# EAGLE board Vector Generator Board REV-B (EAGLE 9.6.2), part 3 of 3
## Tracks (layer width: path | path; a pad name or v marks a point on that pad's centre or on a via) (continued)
XBRM5 (continued)
  Top 0.381: 8C/8D.3 188.59,186.69 188.59,173.74 182.5,167.64 7D.12
XBRM6  (via drill 0.35)
  Top 0.381: v192.79,164.97 182.5,164.97 7D.11
  Bottom 0.381: v192.79,164.97 192.79,150.5 194.69,148.59 8D/8E.4
XBRM7  (via drill 0.35)
  Top 0.381: v174.88,155.83 175.26,156.21 184.4,156.21 | 8D/8E.1 184.4,156.21 | 7D.10 184.4,160.4 184.4,156.21
  Bottom 0.381: v174.88,155.83 174.88,137.16 7E.1
XBRM8
  Top 0.381: 7E.13 192.41,144.78 196.22,144.78 196.98,145.54 196.98,150.88 202.31,150.88 8D/8E.14
XBRM9
  Top 0.381: 7E.12 182.5,132.21 187.45,137.16 196.22,137.16 200.41,141.35 200.41,144.78 203.84,144.78 204.6,145.54 204.6,153.54 202.69,153.54 8D/8E.15
XBRM10
  Top 0.381: 7E.11 182.12,129.54 180.21,131.44 180.21,153.54 194.69,153.54 8D/8E.2
XBRM11  (via drill 0.35)
  Top 0.381: v189.74,127.25 182.5,127.25 7E.10 182.12,127.25 176.02,133.35 172.97,133.35 164.59,141.73 129.54,141.73 v128.78,142.49 | v189.74,150.88 194.69,150.88 8D/8E.3 | v40.39,238.51 52.58,238.51 1B.3 | v87.63,147.83 v40.39,147.83 | v87.63,151.26 102.87,151.26 104.39,152.78 107.82,152.78 113.54,158.5 v128.78,158.5
  Bottom 0.381: v189.74,150.88 v189.74,127.25 | v40.39,147.83 v40.39,238.51 | v87.63,151.26 v87.63,147.83 | v128.78,142.49 v128.78,158.5
XBRMRATE  (via drill 0.35)
  Top 0.381: v187.45,280.42 185.17,278.13 176.02,278.13 174.88,276.99 7A.2 | v192.79,187.83 v187.45,187.83
  Bottom 0.381: v187.45,187.83 v187.45,280.42 | v192.79,187.83 192.79,180.97 194.69,179.07 8C/8D.6
XCUR0  (via drill 0.35)
  Top 0.381: v70.87,230.12 67.06,226.31 55.25,226.31 51.05,222.12 46.48,222.12 45.72,221.36 45.72,214.5 66.68,214.5 | 66.68,214.5 75.44,214.5 80.39,209.55 2C.19 | v128.78,182.5 v161.93,182.5 | v128.78,164.21 128.4,164.59 116.21,164.59 104.78,176.02 v67.82,176.02 | v67.82,212.22 67.44,212.22 66.68,212.98 66.68,214.5
  Bottom 0.381: v70.87,230.12 70.87,241.94 72.77,243.84 2B.1 | v161.93,182.5 6C.9 | v128.78,164.21 v128.78,182.5 | v67.82,212.22 v67.82,176.02
XCUR1  (via drill 0.35)
  Top 0.381: 2C.18 74.3,213.36 v67.82,213.36 | 70.87,238.51 72.77,238.51 2B.3 | 70.87,238.51 v67.82,238.51 | v127.64,181.36 v163.83,181.36 | v116.21,208.41 v127.64,208.41 | v115.06,216.03 114.68,215.65 96.01,215.65 95.63,216.03 92.58,216.03 87.25,221.36 v87.25,221.74 | v87.25,245.36 72.01,245.36 70.87,244.22 70.87,238.51
  Bottom 0.381: v67.82,238.51 v67.82,213.36 | v163.83,181.36 163.83,195.83 162.69,195.83 161.93,196.6 6C.11 | v127.64,208.41 v127.64,181.36 | v116.21,208.41 116.21,214.5 115.06,215.65 v115.06,216.03 | v87.25,245.36 v87.25,221.74
XCUR2  (via drill 0.35)
  Top 0.381: v78.11,224.03 v75.06,224.03 | v159.26,213.74 139.06,213.74 137.16,215.65 116.59,215.65 v116.21,216.03 | v116.21,221.36 115.82,220.98 105.54,220.98 102.87,223.65 83.06,223.65 v81.92,224.79
  Bottom 0.381: 2B.5 75.06,231.65 v75.06,224.03 | 78.11,221.74 78.11,206.88 80.39,204.6 2C.17 | 78.11,221.74 v78.11,224.03 | v159.26,213.74 159.26,206.12 160.4,204.98 160.4,204.6 161.93,204.6 6C.14 | v116.21,221.36 v116.21,216.03 | v81.92,224.79 80.39,223.27 80.39,222.5 79.63,221.74 78.11,221.74
XCUR3  (via drill 0.35)
  Top 0.381: v75.82,203.07 79.25,203.07 80.39,201.93 2C.16 | v79.25,222.88 v75.82,222.88 | v154.31,217.17 129.92,217.17 128.4,218.69 112.01,218.69 v111.63,218.31 | v112.01,228.6 103.63,228.6 102.11,227.08 84.58,227.08 80.77,230.89 2B.9
  Bottom 0.381: v75.82,222.88 v75.82,203.07 | v79.25,222.88 79.25,227.46 78.49,228.22 78.49,228.98 2B.9 | v154.31,217.17 6C.1 | v111.63,218.31 112.01,218.69 v112.01,228.6
XCUR4  (via drill 0.35)
  Top 0.381: v65.53,198.12 74.3,198.12 75.06,198.88 80.01,198.88 80.39,199.26 2C.15 | v65.53,231.65 65.91,232.03 71.25,232.03 71.63,232.41 76.58,232.41 80.39,236.22 2B.11 | 6D.9 159.26,153.54 v143.64,153.54 | v143.64,167.64 119.63,167.64 v119.25,168.02 | v116.97,171.83 115.06,173.74 110.87,173.74 105.16,179.45 v65.53,179.45
  Bottom 0.381: v65.53,231.65 v65.53,198.12 v65.53,179.45 | v143.64,167.64 v143.64,153.54 | v119.25,168.02 116.97,170.31 v116.97,171.83
XCUR5  (via drill 0.35)
  Top 0.381: v148.97,160.02 155.45,160.02 156.21,160.78 161.54,160.78 161.93,161.16 6D.11 | v148.97,214.88 139.06,214.88 137.54,216.41 129.54,216.41 128.02,217.93 112.78,217.93 112.01,217.17 99.06,217.17 96.01,220.22 v94.87,220.22 | v95.25,232.03 94.87,232.41 v82.68,232.41
  Bottom 0.381: 2B.13 82.68,239.27 v82.68,232.41 79.25,232.41 77.72,230.89 77.72,225.55 76.96,224.79 76.96,200.41 80.39,196.98 2C.14 | v148.97,214.88 v148.97,160.02 | v94.87,220.22 94.87,227.46 95.25,227.84 v95.25,232.03
XCUR6  (via drill 0.35)
  Top 0.381: v76.96,172.97 73.15,172.97 2D.1 | v160.4,189.36 160.02,189.74 151.64,189.74 143.26,198.12 v117.73,198.12 | v115.44,198.12 87.25,198.12 83.44,194.31 2C.13
  Bottom 0.381: v76.96,172.97 77.34,173.36 77.34,191.26 80.39,194.31 2C.13 | v160.4,189.36 160.4,179.83 160.02,179.45 160.02,169.93 161.16,169.93 161.93,169.16 6D.14 | v115.44,198.12 v117.73,198.12
XCUR7  (via drill 0.35)
  Top 0.381: v76.2,191.64 80.39,191.64 2C.12 83.06,189.36 v107.44,189.36 | v154.31,185.93 129.16,185.93 v128.78,185.55 | v107.44,201.17 v128.78,201.17
  Bottom 0.381: v76.2,191.64 76.2,183.64 75.82,183.26 75.82,170.31 73.15,167.64 2D.3 | v154.31,185.93 6D.1 | v128.78,201.17 v128.78,185.55 | v107.44,189.36 v107.44,201.17
XCUR8  (via drill 0.35)
  Top 0.381: v73.91,142.49 77.72,138.68 80.39,138.68 2E.19 80.77,138.3 v89.15,138.3 | v139.83,110.11 v161.93,110.11 | v115.82,116.59 v139.45,116.59 | v115.82,140.97 89.54,140.97 v89.15,140.59
  Bottom 0.381: v73.91,142.49 73.91,155.83 75.06,156.97 75.06,160.4 73.15,162.31 2D.5 | v161.93,110.11 6E.9 | v139.83,110.11 139.45,110.49 v139.45,116.59 | v115.82,140.97 v115.82,116.59 | v89.15,138.3 v89.15,140.59
XCUR9  (via drill 0.35)
  Top 0.381: 6E.11 153.92,117.73 v101.73,117.73 | v91.44,112.01 v101.73,112.01 | v91.44,126.87 91.44,129.16 84.96,135.64 80.77,135.64 2E.18
  Bottom 0.381: 2E.18 80.39,136.02 78.49,137.92 78.49,152.78 82.68,156.97 82.68,158.12 80.77,160.02 2D.9 | v101.73,112.01 v101.73,117.73 | v91.44,126.87 v91.44,112.01
XCUR10  (via drill 0.35)
  Top 0.381: v76.58,136.02 77.72,136.02 80.39,133.35 2E.17 86.11,133.35 90.3,129.16 v90.3,126.87 | v76.96,164.97 80.39,164.97 2D.11 | v100.58,118.87 v153.54,118.87
  Bottom 0.381: v76.58,136.02 76.96,136.4 v76.96,164.97 | 6E.14 159.64,131.06 159.64,129.54 156.21,126.11 156.21,120.02 155.07,118.87 v153.54,118.87 | v100.58,118.87 100.58,105.16 94.49,99.06 90.3,99.06 v90.3,126.87
XCUR11  (via drill 0.35)
  Top 0.381: v75.44,134.87 76.58,134.87 2E.16 80.77,131.06 v85.73,131.06 | v75.82,168.78 76.96,169.93 80.39,169.93 2D.13 | v128.78,140.97 152.02,140.97 154.31,138.68 6E.1 | v127.64,148.21 127.25,148.59 90.3,148.59 88.77,150.11 v85.73,150.11
  Bottom 0.381: v75.44,134.87 75.44,139.83 76.2,140.59 76.2,164.21 75.82,164.59 v75.82,168.78 | v128.78,140.97 127.64,142.11 v127.64,148.21 | v85.73,131.06 v85.73,150.11
XEND0  (via drill 0.35)
  Top 0.381: v86.87,190.5 97.16,190.5 3C.10 v115.44,194.31 | v62.48,185.17 v86.87,185.17 | v241.55,195.45 241.17,195.45 241.17,193.93 243.08,192.02 10C.9 | v239.65,212.6 239.27,212.22 221.36,212.22 220.6,211.46 220.6,207.26 | 220.6,207.26 222.88,207.26 9C.15 | v194.31,194.31 6C.10 | 220.6,207.26 219.07,205.74 214.12,205.74 212.98,206.88 v194.31,206.88 190.12,211.07 146.69,211.07 v143.64,208.03 | v117.73,192.79 118.49,192.02 131.06,192.02 132.59,190.5 135.25,190.5 139.45,194.69 v139.45,196.98
  Top 0.432: 1C.19 2C.2
  Bottom 0.381: v86.87,185.17 v86.87,190.5 | v62.48,185.17 62.48,207.65 60.58,209.55 1C.19 | v241.55,195.45 239.65,197.36 v239.65,212.6 | v194.31,206.88 v194.31,194.31 | v115.44,194.31 116.97,192.79 v117.73,192.79 | v139.45,196.98 139.45,197.36 140.21,198.12 143.64,198.12 v143.64,208.03
XEND1  (via drill 0.35)
  Top 0.381: v83.06,192.02 93.34,192.02 | v83.06,205.74 74.3,205.74 2C.3 | 211.84,212.98 v160.4,212.98 160.4,214.12 158.5,216.03 v139.45,216.03 | 9C.1 211.84,212.98 | v240.79,213.74 212.6,213.74 211.84,212.98 | 93.34,192.02 94.11,192.79 97.92,192.79 v98.3,193.17 | v108.59,190.5 v98.68,190.5 | v131.83,204.6 v108.59,204.6 | 93.34,192.02 3C.8
  Top 0.432: 2C.3 1C.18
  Bottom 0.381: v83.06,205.74 v83.06,192.02 | v160.4,212.98 160.02,212.6 160.02,206.5 160.78,205.74 163.07,205.74 163.83,204.98 163.83,200.41 162.69,200.41 161.93,199.64 6C.12 | 10C.11 240.41,199.64 240.41,211.84 240.79,212.22 v240.79,213.74 | v98.3,193.17 98.68,192.79 v98.68,190.5 | v108.59,204.6 v108.59,190.5 | v131.83,204.6 131.83,209.93 137.92,216.03 v139.45,216.03
XEND2  (via drill 0.35)
  Top 0.381: v75.06,184.02 v96.01,184.02 97.92,185.93 111.63,185.93 112.4,186.69 v124.97,186.69 | v240.41,225.93 v228.22,225.93 v158.12,225.93 | v228.22,194.31 9C.10 | v159.26,180.21 v124.97,180.21
  Top 0.432: 1C.17 2C.4
  Bottom 0.381: v96.01,184.02 96.39,184.4 96.39,204.6 93.34,204.6 3C.3 | v75.06,184.02 75.06,202.31 73.15,204.22 2C.4 | 159.26,204.6 158.12,205.74 v158.12,225.93 | 159.26,204.6 6C.13 | v240.41,225.93 240.41,215.65 241.94,214.12 241.94,210.69 241.17,209.93 241.17,206.5 10C.14 | v228.22,225.93 v228.22,194.31 | v124.97,180.21 v124.97,186.69 | 159.26,204.6 v159.26,180.21
XEND3  (via drill 0.35)
  Top 0.381: v88.39,209.17 92.96,209.17 | v73.53,217.17 v86.49,217.17 | 9C.9 222.88,192.02 223.65,192.79 228.6,192.79 233.93,198.12 236.98,198.12 238.51,199.64 238.51,208.03 237.36,208.03 235.84,209.55 10C.1 | v169.55,207.26 161.93,207.26 6C.15 | v235.46,214.88 v169.55,214.88 | 92.96,209.17 96.77,209.17 97.54,208.41 v97.54,206.12 | v128.78,203.45 v104.01,203.45 | v128.78,224.03 129.16,223.65 v169.55,223.65 | 92.96,209.17 3C.1
  Top 0.432: 2C.5 1C.16
  Bottom 0.381: v88.39,209.17 86.49,211.07 v86.49,217.17 | v73.53,217.17 75.06,215.65 75.06,206.5 74.3,205.74 70.87,205.74 70.87,203.84 72.77,201.93 2C.5 | v169.55,207.26 v169.55,214.88 v169.55,223.65 | v235.46,214.88 235.46,209.55 10C.1 | v97.54,206.12 99.06,207.65 99.06,210.31 99.82,211.07 104.01,211.07 v104.01,203.45 | v128.78,224.03 v128.78,203.45
XEND4  (via drill 0.35)
  Top 0.381: 10D.9 241.17,156.21 241.17,163.45 236.98,167.64 234.31,167.64 233.17,168.78 225.55,168.78 9D.15 217.55,176.78 217.55,177.93 212.98,177.93 207.65,172.59 v189.74,172.59 | 104.39,162.31 100.97,158.88 3D.10 | v127.64,162.31 104.39,162.31 | v127.64,151.26 160.4,151.26 163.83,154.69 | 163.83,154.69 163.83,158.5 161.93,158.5 6D.10 | v70.87,190.5 70.87,187.07 v102.87,187.07 | v102.87,165.35 104.39,163.83 104.39,162.31 | 163.83,154.69 v189.74,154.69
  Top 0.432: 1C.15 2C.6
  Bottom 0.381: v127.64,151.26 v127.64,162.31 | v70.87,190.5 70.87,197.36 72.77,199.26 2C.6 | v102.87,165.35 v102.87,187.07 | v189.74,154.69 v189.74,172.59
XEND5  (via drill 0.35)
  Top 0.381: 3D.8 95.25,158.12 95.63,158.12 99.06,161.54 99.06,166.88 99.44,167.26 v99.44,167.64 107.82,167.64 112.01,163.45 128.02,163.45 129.54,161.93 v131.83,161.93 | v58.29,177.17 v99.06,177.17 | v164.21,171.45 176.02,171.45 180.21,167.26 180.21,163.83 v188.59,163.83 v212.98,163.83 | v240.03,115.44 240.41,115.44 241.17,114.68 241.17,113.16 219.84,113.16 219.07,113.92 v188.59,113.92 | v163.83,150.11 v136.02,150.11
  Top 0.432: 2C.7 1C.14
  Bottom 0.381: v99.44,167.64 99.44,168.02 99.06,168.4 v99.06,177.17 | v58.29,177.17 58.29,194.69 60.2,196.6 1C.14 | 163.83,165.74 164.21,166.12 v164.21,171.45 | 163.83,165.74 6D.12 | v212.98,163.83 213.36,164.21 213.36,172.21 215.26,174.12 9D.1 | 10D.11 240.03,158.12 v240.03,115.44 | v188.59,163.83 v188.59,113.92 | v131.83,161.93 131.83,160.78 132.59,160.02 136.02,160.02 v136.02,150.11 | 163.83,165.74 v163.83,150.11
XEND6  (via drill 0.35)
  Top 0.381: v85.73,198.12 76.96,198.12 73.15,194.31 2C.8 | v228.22,158.88 222.88,158.88 9D.10 | v228.22,116.59 228.6,116.97 238.51,116.97 v238.89,116.59 | v164.21,105.16 228.22,105.16 230.12,103.25 v233.17,103.25 | v104.78,154.69 91.44,154.69 91.44,166.88 93.34,168.78 3D.3 | v104.78,151.64 105.16,152.02 108.2,152.02 112.4,156.21 130.3,156.21 134.11,152.4 v160.02,152.4
  Top 0.432: 1C.13 2C.8
  Bottom 0.381: v85.73,198.12 85.73,174.12 90.68,169.16 93.34,169.16 3D.3 | v228.22,116.59 v228.22,158.88 | 10D.14 239.27,164.97 239.27,116.97 v238.89,116.59 238.89,116.97 237.36,116.97 236.6,116.2 236.6,106.68 v233.17,103.25 | v164.21,105.16 164.59,105.54 164.59,137.16 160.78,137.16 160.02,137.92 v160.02,152.4 160.02,165.35 161.16,165.35 161.93,166.12 6D.13 | v104.78,151.64 v104.78,154.69
XEND7  (via drill 0.35)
  Top 0.381: v93.34,188.21 92.96,187.83 76.96,187.83 2C.9 | v233.55,157.73 224.41,157.73 9D.9 221.36,154.69 214.12,154.69 211.07,157.73 v187.45,157.73 | 6D.15 165.35,174.88 178.31,174.88 | 178.31,174.88 184.02,174.88 184.4,175.26 v187.45,175.26 | v93.34,178.31 105.16,178.31 110.87,172.59 v114.68,172.59 | v119.25,179.07 139.06,179.07 140.21,177.93 176.78,177.93 178.31,176.4 178.31,174.88
  Top 0.432: 2C.9 1C.12
  Bottom 0.381: v93.34,188.21 v93.34,178.31 3D.1 | v233.55,157.73 233.55,171.83 235.46,173.74 10D.1 | v187.45,157.73 v187.45,175.26 | v114.68,172.59 119.25,177.17 v119.25,179.07
XEND8  (via drill 0.35)
  Top 0.381: v75.06,155.45 74.3,156.21 66.68,156.21 1D.15 | v224.79,119.63 225.17,119.25 240.79,119.25 241.94,120.4 243.08,120.4 10E.9 | 98.3,114.3 98.3,113.16 163.07,113.16 v163.45,113.54 | 98.3,114.3 98.3,120.4 100.97,123.06 3E.10 | v163.45,107.06 v224.79,107.06 | v66.68,138.3 72.77,138.3 2E.2 | 98.3,114.3 v66.68,114.3
  Bottom 0.381: v75.06,155.45 75.06,140.59 73.15,138.68 2E.2 | 9E.15 222.88,135.64 223.65,134.87 224.79,134.87 v224.79,119.63 v224.79,107.06 | 6E.10 161.93,123.06 163.83,121.16 163.83,113.92 v163.45,113.54 v163.45,107.06 | v66.68,114.3 v66.68,138.3
XEND9  (via drill 0.35)
  Top 0.381: v77.34,121.92 81.92,121.92 82.68,121.16 92.96,121.16 93.34,120.78 3E.8 | v56.39,136.02 72.77,136.02 2E.3 | 197.36,129.54 206.12,138.3 215.26,138.3 9E.1 | 197.36,129.54 188.21,120.4 172.59,120.4 165.74,127.25 162.69,127.25 161.93,128.02 6E.12 | v245.36,112.78 244.98,112.4 219.07,112.4 v218.69,112.78 | 197.36,129.54 v217.93,129.54 | v93.34,110.87 139.06,110.87 139.45,111.25 v160.4,111.25
  Bottom 0.381: v77.34,121.92 76.58,122.68 76.58,132.21 73.15,135.64 2E.3 | v56.39,136.02 56.39,156.21 60.2,160.02 1D.14 | v245.36,112.78 245.36,123.83 243.46,125.73 10E.11 | v218.69,112.78 218.31,113.16 218.31,129.16 v217.93,129.54 | v93.34,110.87 3E.8 | v160.4,111.25 160.4,119.63 160.02,120.02 160.02,126.49 161.93,128.4 6E.12
XEND10  (via drill 0.35)
  Top 0.381: v57.53,133.35 2E.4 | v96.01,119.25 96.01,118.87 93.73,116.59 v76.2,116.59 | 219.07,119.25 v159.26,119.25 156.97,116.97 140.97,116.97 v140.59,116.59 | 219.07,119.25 222.88,123.06 9E.10 | v241.55,118.49 219.84,118.49 219.07,119.25 | v96.01,108.97 96.39,109.35 137.54,109.35 v137.92,108.97
  Bottom 0.381: v57.53,133.35 57.53,155.83 59.06,157.35 60.2,157.35 1D.13 | 3E.3 96.01,130.68 v96.01,119.25 v96.01,108.97 | v76.2,116.59 75.82,116.97 75.82,130.68 73.15,133.35 2E.4 | v159.26,119.25 159.26,128.02 161.93,130.68 6E.13 | v241.55,118.49 241.17,118.87 241.17,131.44 243.08,133.35 10E.14 | v137.92,108.97 138.3,109.35 138.3,116.97 139.06,117.73 140.59,117.73 v140.59,116.59
XEND11  (via drill 0.35)
  Top 0.381: 91.44,137.16 92.2,137.16 93.34,138.3 3E.1 | 91.44,137.16 v70.87,137.16 v62.48,137.16 | 160.02,129.54 160.02,134.11 160.78,134.87 161.16,134.87 161.93,135.64 6E.15 | 160.02,129.54 164.59,129.54 168.4,125.73 192.41,125.73 207.26,140.59 228.6,140.59 228.98,140.97 233.17,140.97 235.46,138.68 10E.1 | v237.36,121.92 224.03,121.92 222.88,120.78 9E.9 | 91.44,137.16 91.44,130.3 92.2,129.54 105.16,129.54 112.78,121.92 155.45,121.92 160.02,126.49 160.02,129.54
  Bottom 0.381: 2E.5 70.87,132.97 v70.87,137.16 | 1D.12 62.48,152.78 v62.48,137.16 | v237.36,121.92 237.74,122.3 237.74,136.4 235.84,138.3 10E.1
XOUT
  Top 0.381: VR1.3 315.47,157.35 313.18,157.35 VR1.2
  Bottom 0.381: IC11.1 313.18,150.11 313.18,157.35 VR1.2 313.18,157.73 313.18,167.64 C41.1 | X1.6 319.66,130.68 319.66,153.54 315.85,157.35 VR1.3
XRATE  (via drill 0.35)
  Top 0.381: v209.93,270.51 183.64,270.51 182.5,271.65 7A.11 | v208.79,198.12 216.41,198.12 219.46,201.17 219.46,204.22 222.88,204.22 9C.14
  Bottom 0.381: 9E.14 220.98,135.25 220.98,151.64 224.79,155.45 224.79,166.88 222.88,168.78 | 222.88,168.78 220.98,170.69 220.98,174.5 224.79,178.31 224.79,203.45 223.65,203.45 222.88,204.22 9C.14 | 222.88,168.78 9D.14 | v209.93,270.51 209.93,220.98 208.79,219.84 v208.79,198.12
YBRM0  (via drill 0.35)
  Top 0.381: v198.5,99.06 7F.13
  Bottom 0.381: v198.5,99.06 198.5,90.3 196.98,88.77 196.98,79.63 195.07,77.72 8F/8G.4
YBRM1  (via drill 0.35)
  Top 0.381: v184.79,84.96 194.69,84.96 8F/8G.1
  Bottom 0.381: v184.79,84.96 184.4,85.34 184.4,94.49 182.5,96.39 7F.12
YBRM2  (via drill 0.35)
  Top 0.381: 7F.11 185.17,91.06 v201.17,91.06
  Bottom 0.381: v201.17,91.06 200.79,90.68 200.79,85.72 200.41,85.34 200.41,81.91 202.31,80.01 8F/8G.14
YBRM3
  Top 0.381: 192.41,83.82 7G.1 | 192.41,83.82 201.17,83.82 202.31,82.68 8F/8G.15 | 192.41,83.82 183.64,83.82 183.64,85.34 184.4,86.11 184.4,89.53 182.5,91.44 7F.10
YBRM4
  Top 0.381: 7G.13 182.5,63.63 192.02,73.15 192.02,82.3 194.69,82.3 8F/8G.2
YBRM5
  Top 0.381: 8F/8G.3 192.79,80.01 192.79,71.25 182.5,60.96 7G.12
YBRM6
  Top 0.381: 8G/8H.4 188.59,41.91 188.59,44.58 189.36,45.34 189.74,45.34 189.74,56.39 188.21,57.91 182.88,57.91 182.5,58.29 7G.11
YBRM7  (via drill 0.35)
  Top 0.381: v184.79,32.77 177.17,32.77 174.88,30.48 7H.1 | v184.4,59.05 190.5,59.05 190.5,53.72 194.69,49.53 8G/8H.1
  Bottom 0.381: v184.79,32.77 184.4,33.15 184.4,53.72 | 7G.10 184.4,53.72 | 184.4,53.72 v184.4,59.05
YBRM8
  Top 0.381: 7H.13 184.79,30.48 196.22,30.48 200.41,34.67 200.41,44.2 202.31,44.2 8G/8H.14
YBRM9  (via drill 0.35)
  Top 0.381: v205.36,27.05 184.02,27.05 182.5,25.53 7H.12
  Bottom 0.381: v205.36,27.05 205.36,44.2 8G/8H.15
YBRM10
  Top 0.381: 7H.11 182.12,22.86 180.21,24.77 180.21,32 184.02,32 184.4,31.62 187.83,31.62 192.79,36.58 192.79,38.1 196.22,38.1 196.98,38.86 196.98,46.86 195.07,46.86 8G/8H.2
YBRM11  (via drill 0.35)
  Top 0.381: v189.74,44.2 194.69,44.2 8G/8H.3 | v34.67,241.17 52.58,241.17 1B.2 | v34.67,19.05 65.53,19.05 75.06,9.52 135.64,9.52 138.3,6.86 184.02,6.86 v184.4,7.24
  Bottom 0.381: 184.4,22.48 187.45,25.53 187.45,41.91 v189.74,44.2 | 184.4,22.48 7H.10 | v34.67,19.05 v34.67,241.17 | 184.4,22.48 v184.4,7.24
YBRMRATE  (via drill 0.35)
  Top 0.381: v208.03,128.02 v197.36,128.02 | v208.79,249.56 179.83,249.56 176.78,246.51 176.78,241.55 174.88,241.55 7B.2
  Bottom 0.381: v197.36,128.02 197.36,98.68 197.74,98.3 197.74,92.2 192.79,87.25 192.79,74.3 194.69,72.39 8F/8G.6 | v208.03,128.02 208.03,140.59 208.79,141.35 208.79,177.17 210.31,178.69 210.31,192.41 207.65,195.07 207.65,239.27 208.79,240.41 v208.79,249.56
YCUR0  (via drill 0.35)
  Top 0.381: v67.82,101.73 72.77,101.73 2F.1 | v67.82,129.54 79.25,129.54 80.39,128.4 2E.15 | v127.64,76.58 131.06,76.58 136.78,82.3 159.26,82.3 161.93,84.96 6F.9 | v115.44,53.34 v127.64,53.34 | v67.82,81.53 v110.49,81.53
  Bottom 0.381: v67.82,129.54 v67.82,101.73 v67.82,81.53 | v127.64,53.34 v127.64,76.58 | v115.44,53.34 115.82,53.72 115.82,71.63 115.06,72.39 110.49,72.39 v110.49,81.53
YCUR1  (via drill 0.35)
  Top 0.381: v85.73,102.49 85.34,102.87 79.25,102.87 73.15,96.77 2F.3 | 2E.14 v85.73,125.73 | v156.97,106.3 128.4,106.3 128.02,105.92 v124.97,105.92 | v121.92,105.92 91.06,105.92 90.3,105.16 v88.01,105.16
  Bottom 0.381: v85.73,125.73 85.73,105.16 | 85.73,105.16 v85.73,102.49 | v156.97,106.3 156.97,95.25 161.93,90.3 6F.11 | v121.92,105.92 v124.97,105.92 | 85.73,105.16 v88.01,105.16
YCUR2  (via drill 0.35)
  Top 0.381: v70.87,115.44 93.73,115.44 v97.16,118.87 97.16,121.92 83.06,121.92 81.92,123.06 80.77,123.06 2E.13 | v99.44,115.44 v159.26,115.44
  Bottom 0.381: v70.87,115.44 70.87,93.34 72.77,91.44 2F.5 | v159.26,115.44 159.26,100.58 161.93,97.92 6F.14 | v99.44,115.44 97.16,117.73 v97.16,118.87
YCUR3  (via drill 0.35)
  Top 0.381: 2F.9 78.49,91.06 v78.49,93.34 | v99.44,114.3 v154.31,114.3 | v94.87,119.25 81.92,119.25 80.77,120.4 2E.12
  Bottom 0.381: v78.49,93.34 78.49,118.49 2E.12 | v154.31,114.3 6F.1 | v99.44,114.3 97.16,112.01 97.16,108.59 96.39,107.82 94.87,107.82 v94.87,119.25
YCUR4  (via drill 0.35)
  Top 0.381: 6G.9 158.12,45.72 127.64,45.72 123.06,50.29 v116.97,50.29 | v116.59,72.39 97.54,72.39 96.77,73.15 88.77,73.15 83.06,78.87 v78.11,78.87
  Bottom 0.381: 2F.11 78.11,91.44 v78.11,78.87 78.11,69.72 80.39,67.44 2G.19 | v116.97,50.29 116.59,50.67 v116.59,72.39
YCUR5  (via drill 0.35)
  Top 0.381: v75.44,97.54 76.96,99.06 2F.13 | v144.02,52.2 145.54,52.2 146.69,53.34 160.78,53.34 161.93,54.48 6G.11 | v142.49,34.29 117.35,34.29 v116.97,33.91 | v82.68,39.24 v110.87,39.24
  Bottom 0.381: v75.44,97.54 75.44,82.3 76.96,80.77 76.96,68.2 80.39,64.77 2G.18 80.77,64.77 82.68,62.87 v82.68,39.24 | v144.02,52.2 143.64,51.82 143.64,35.43 v142.49,34.29 | v116.97,33.91 115.44,33.91 115.06,34.29 110.87,34.29 v110.87,39.24
YCUR6  (via drill 0.35)
  Top 0.381: v65.53,30.48 2H.1 73.15,30.48 76.58,33.91 108.97,33.91 v109.35,34.29 | v65.53,68.58 74.3,68.58 2G.17 | v167.26,62.48 161.93,62.48 6G.14 | v123.44,73.15 v167.26,73.15 | v123.44,62.87 123.06,62.48 112.01,62.48 v109.35,59.82
  Bottom 0.381: v65.53,68.58 v65.53,30.48 | v167.26,73.15 v167.26,62.48 | v123.44,62.87 v123.44,73.15 | v109.35,34.29 v109.35,59.82
YCUR7  (via drill 0.35)
  Top 0.381: 77.72,51.05 v75.06,51.05 | 77.72,51.05 78.49,51.82 78.49,59.44 80.39,59.44 2G.16 | v152.4,51.05 149.35,48.01 v137.16,48.01 | v123.44,40.01 v137.16,40.01 | v119.25,39.62 116.97,41.91 96.39,41.91 93.73,44.58 80.39,44.58 77.72,47.24 77.72,51.05
  Bottom 0.381: 2H.3 75.06,27.43 v75.06,51.05 | v152.4,51.05 152.4,66.29 153.54,66.29 154.31,67.06 6G.1 | v137.16,40.01 v137.16,48.01 | v123.44,40.01 123.44,35.05 122.68,34.29 119.25,34.29 v119.25,39.62
YCUR8  (via drill 0.35)
  Top 0.381: v139.45,9.52 v161.93,9.52 | v75.06,7.24 v136.4,7.24 | v66.68,53.34 v77.34,53.34 | v66.68,20.57 72.77,20.57 2H.5
  Bottom 0.381: v161.93,9.52 6H.9 | v139.45,9.52 137.16,7.24 v136.4,7.24 | v75.06,7.24 75.06,18.29 2H.5 | v77.34,53.34 77.34,54.1 80.39,57.15 2G.15 | v66.68,20.57 v66.68,53.34
YCUR9  (via drill 0.35)
  Top 0.381: 2H.9 85.73,22.86 v90.3,22.86 102.11,22.86 103.25,24 v131.83,24 | v88.39,54.48 80.77,54.48 2G.14 | 6H.11 158.12,15.24 140.21,15.24 v139.45,14.48
  Bottom 0.381: v90.3,22.86 88.39,24.77 v88.39,54.48 | v139.45,14.48 139.45,13.34 140.59,12.19 140.59,11.43 139.83,10.67 136.02,10.67 136.02,14.48 135.25,15.24 131.83,15.24 v131.83,24
YCUR10  (via drill 0.35)
  Top 0.381: v85.73,51.82 80.77,51.82 2G.13 | 2H.11 80.39,22.86 77.72,25.53 76.96,25.53 76.2,26.29 76.2,30.1 77.72,30.1 79.63,32 85.34,32 v85.73,31.62 89.92,31.62 91.44,33.15 103.25,33.15 106.68,29.72 118.49,29.72 118.87,29.34 125.73,29.34 v126.11,28.96 | 6H.14 158.12,30.48 151.26,30.48 144.4,37.34 v126.11,37.34
  Bottom 0.381: v85.73,51.82 v85.73,31.62 | v126.11,28.96 v126.11,37.34
YCUR11  (via drill 0.35)
  Top 0.381: v116.97,49.15 117.35,49.15 117.73,49.53 122.68,49.53 130.3,41.91 139.06,41.91 140.21,40.77 142.11,40.77 146.3,36.58 149.73,36.58 154.31,32 6H.1 | v111.63,44.96 111.25,45.34 84.96,45.34 80.77,49.53 2G.12
  Bottom 0.381: 2H.13 78.49,30.1 78.49,47.62 80.39,49.53 2G.12 | v116.97,49.15 116.97,43.81 115.06,41.91 111.63,41.91 v111.63,44.96
YEND0  (via drill 0.35)
  Top 0.381: v76.58,82.68 96.01,82.68 3F.10 101.73,88.39 v117.35,88.39 | v76.58,104.78 62.48,104.78 60.58,102.87 1F.19 | v163.83,101.35 166.88,104.39 218.69,104.39 222.5,100.58 222.88,100.58 9F.15 222.88,100.2 224.03,100.2 225.17,99.06 237.74,99.06 237.74,90.68 243.08,85.34 10F.9 | v123.44,74.3 123.83,74.68 136.4,74.68 143.26,81.53 160.78,81.53 163.83,84.58 163.83,87.63 6F.10
  Bottom 0.381: v76.58,82.68 v76.58,104.78 76.58,114.68 75.06,116.2 75.06,126.11 73.15,128.02 2E.6 | 6F.10 163.83,89.53 v163.83,101.35 | v117.35,88.39 119.25,86.49 119.25,80.77 120.02,80.01 123.44,80.01 v123.44,74.3
YEND1  (via drill 0.35)
  Top 0.381: v62.48,84.96 93.34,84.96 3F.8 93.34,85.34 94.11,86.11 94.49,86.11 99.82,91.44 113.16,91.44 114.68,92.96 v120.78,92.96 | v58.29,125.73 2E.7 | 9F.1 v209.93,102.87 180.21,102.87 180.21,99.44 176.02,95.25 173.36,95.25 171.83,93.73 162.69,93.73 161.93,92.96 6F.12 | v240.03,114.3 239.65,113.92 220.22,113.92 219.46,114.68 210.31,114.68 v209.93,115.06 170.31,115.06 167.64,112.4 121.16,112.4 v120.78,112.01
  Bottom 0.381: v62.48,84.96 62.48,98.3 60.58,100.2 1F.18 60.2,100.58 58.29,102.49 v58.29,125.73 | 10F.11 240.03,93.34 v240.03,114.3 | v209.93,102.87 v209.93,115.06 | v120.78,112.01 v120.78,92.96
YEND2  (via drill 0.35)
  Top 0.381: 86.87,103.63 87.63,103.63 93.34,97.92 3F.3 | 86.87,103.63 66.29,103.63 60.58,97.92 1F.17 | v57.15,123.06 72.77,123.06 2E.8 | 86.87,103.63 86.87,105.54 87.63,106.3 90.3,106.3 94.11,110.11 138.3,110.11 139.45,108.97 v158.12,108.97 162.31,108.97 163.45,110.11 187.07,110.11 v187.45,110.49 v249.56,110.49 | 9F.10 219.07,83.82 206.5,83.82 203.84,86.49 v187.45,86.49 | v249.56,97.92 243.46,97.92 10F.14
  Bottom 0.381: v57.15,123.06 57.53,122.68 57.53,100.58 1F.17 | 6F.13 158.12,99.06 v158.12,108.97 | v187.45,110.49 v187.45,86.49 | v249.56,110.49 v249.56,97.92
YEND3  (via drill 0.35)
  Top 0.381: 58.29,109.73 58.29,120.4 72.77,120.4 2E.9 | 58.29,109.73 58.29,97.16 60.2,95.25 1F.16 | v237.74,84.2 237.36,84.2 236.98,83.82 234.31,83.82 233.93,84.2 223.65,84.2 222.88,84.96 9F.9 222.88,85.34 223.65,86.11 224.03,86.11 224.79,86.87 224.79,91.44 219.46,91.44 218.31,90.3 217.55,90.3 216.41,91.44 204.6,91.44 200.79,95.25 v177.93,95.25 | 3F.1 94.87,104.39 102.11,104.39 102.49,104.01 124.59,104.01 125.73,105.16 128.4,105.16 128.78,105.54 154.31,105.54 158.5,101.35 161.16,101.35 161.93,100.58 6F.15 161.93,100.2 164.21,100.2 166.88,102.87 v177.93,102.87 | v92.2,109.73 58.29,109.73
  Bottom 0.381: v237.74,84.2 237.74,100.97 235.84,102.87 10F.1 | v177.93,102.87 v177.93,95.25 | v92.2,109.73 93.34,108.59 3F.1
YEND4  (via drill 0.35)
  Top 0.381: v62.48,40.77 v102.87,40.77 | 162.69,51.05 161.93,51.82 6G.10 | 162.69,51.05 171.83,51.05 173.36,49.53 v187.45,49.53 | v187.45,60.96 219.07,60.96 9G.15 | v225.17,45.72 v238.51,45.72 | v103.25,27.43 126.87,27.43 127.25,27.81 v128.78,27.81 | v128.78,46.86 156.59,46.86 160.78,51.05 162.69,51.05
  Top 0.432: 1G.19 2G.2
  Bottom 0.381: v62.48,40.77 62.48,65.15 1G.19 | 3G.10 100.97,51.82 101.73,51.05 102.87,51.05 v102.87,40.77 103.25,40.39 v103.25,27.43 | v187.45,60.96 v187.45,49.53 | v238.51,45.72 239.27,45.72 243.08,49.53 10G.9 | v225.17,45.72 225.55,46.1 225.55,62.1 9G.15 | v128.78,46.86 v128.78,27.81
YEND5  (via drill 0.35)
  Top 0.381: 3G.8 96.01,52.2 96.01,70.48 | 96.01,70.48 96.01,71.25 64.39,71.25 61.72,68.58 59.06,68.58 58.29,67.82 58.29,64.77 1G.18 | 6G.12 187.45,57.15 v188.59,56.01 | v188.98,65.91 213.74,65.91 214.88,67.06 215.26,67.06 9G.1 215.26,67.44 217.17,69.34 237.36,69.34 v237.74,68.96 | v96.77,70.48 96.01,70.48 | v128.78,94.11 v102.87,94.11 | v158.88,71.63 v128.78,71.63
  Top 0.432: 1G.18 2G.3
  Bottom 0.381: v188.59,56.01 188.98,56.39 v188.98,65.91 | v237.74,68.96 238.89,67.82 238.89,59.05 243.08,54.86 10G.11 | v96.77,70.48 96.77,96.01 99.82,99.06 102.87,99.06 v102.87,94.11 | v128.78,71.63 v128.78,94.11 | v158.88,71.63 158.88,60.2 6G.12
YEND6  (via drill 0.35)
  Top 0.381: 2G.4 74.3,60.96 81.92,60.96 82.68,61.72 92.96,61.72 93.34,62.1 3G.3 | v192.79,40.77 v163.83,40.77 | v192.79,53.34 220.6,53.34 221.74,52.2 222.88,52.2 | 10G.14 241.94,60.96 v229.36,60.96 | 222.88,52.2 v229.36,52.2 | 222.88,52.2 9G.10 | v107.44,60.96 v97.16,60.96 | v131.83,56.01 v107.44,56.01 | v160.02,70.48 v131.83,70.48
  Top 0.432: 2G.4 1G.17
  Bottom 0.381: v163.83,40.77 163.83,58.67 162.69,58.67 161.93,59.44 6G.13 161.93,59.82 160.02,61.72 v160.02,70.48 | v192.79,53.34 v192.79,40.77 | v229.36,52.2 v229.36,60.96 | v97.16,60.96 97.16,62.1 93.34,62.1 3G.3 | v107.44,56.01 v107.44,60.96 | v131.83,70.48 v131.83,56.01
YEND7  (via drill 0.35)
  Top 0.381: v75.82,68.58 92.2,68.58 93.34,67.44 3G.1 | v169.55,64.77 6G.15 | v169.55,108.97 169.93,109.35 230.12,109.35 v230.5,108.97 | v230.5,67.44 235.46,67.44 10G.1 | v230.5,49.53 9G.9 | v90.3,77.72 v93.34,74.68 | v90.3,91.44 94.49,91.44 99.06,96.01 99.06,99.06 135.25,99.06 140.59,104.39 v147.83,104.39 | v169.55,78.11 v147.83,78.11
  Top 0.432: 1G.16 2G.5
  Bottom 0.381: v75.82,68.58 75.06,67.82 75.06,61.72 2G.5 | v169.55,108.97 v169.55,78.11 v169.55,64.77 | v230.5,108.97 v230.5,67.44 v230.5,49.53 | v93.34,74.68 3G.1 | v90.3,91.44 v90.3,77.72 | v147.83,78.11 v147.83,104.39
YEND8  (via drill 0.35)
  Top 0.381: 10H.9 241.94,15.24 v224.79,15.24 184.79,15.24 183.26,13.72 v178.69,13.72 | v137.16,15.24 132.59,15.24 131.44,16.38 100.97,16.38 3H.10 | v139.45,11.81 157.35,11.81 158.12,12.57 | 158.12,12.57 161.93,16.38 6H.10 | v99.06,8.38 v67.82,8.38 | 158.12,12.57 v176.4,12.57
  Top 0.432: 2G.6 v67.82,57.15 1G.15
  Bottom 0.381: v224.79,15.24 224.79,28.19 223.65,28.19 222.88,28.96 9H.15 | v137.16,15.24 138.68,13.72 138.68,12.57 v139.45,11.81 | v67.82,8.38 v67.82,57.15 | v99.06,8.38 99.06,14.48 100.97,16.38 3H.10 | v178.69,13.72 177.55,12.57 v176.4,12.57
YEND9  (via drill 0.35)
  Top 0.381: v78.49,13.72 93.34,13.72 3H.8 | v176.4,16.76 176.78,16.76 176.78,18.29 176.02,19.05 173.36,19.05 171.83,20.57 162.69,20.57 161.93,21.34 6H.12 | v179.45,19.05 202.69,19.05 215.26,31.62 9H.1 215.26,32 217.17,33.91 229.74,33.91 230.12,34.29 238.89,34.29 238.89,32.77 238.51,32.39 v238.51,31.24 | v131.83,25.53 v102.87,25.53 | v160.02,44.2 v131.83,44.2
  Top 0.432: 1G.14 2G.7
  Bottom 0.381: v78.49,13.72 76.2,16 76.2,51.44 2G.7 | v176.4,16.76 178.69,19.05 v179.45,19.05 | v238.51,31.24 238.51,23.62 243.08,19.05 10H.11 | v102.87,25.53 102.87,22.86 99.82,22.86 97.54,20.57 97.54,14.1 93.34,14.1 3H.8 | v131.83,44.2 v131.83,25.53 | v160.02,44.2 160.02,31.24 160.78,30.48 163.83,30.48 163.83,23.62 161.93,21.72 6H.12
YEND10  (via drill 0.35)
  Top 0.381: v233.17,16.38 222.88,16.38 9H.10 | v139.83,22.86 155.45,22.86 156.59,24 161.93,24 6H.13 161.93,24.38 164.59,24.38 174.12,33.91 v188.59,33.91 | v104.39,22.86 v136.02,22.86 | v104.39,30.48 99.82,30.48 96.01,26.67 3H.3 v77.34,26.67 | v77.34,52.2 73.15,52.2 2G.8 | v237.74,11.05 188.98,11.05 v188.59,10.67
  Top 0.432: 2G.8 1G.13
  Bottom 0.381: v233.17,16.38 234.31,15.24 237.74,15.24 | 237.74,15.24 245.36,15.24 245.36,24.77 243.46,26.67 10H.14 | v136.02,22.86 v139.83,22.86 | v104.39,30.48 v104.39,22.86 | v77.34,26.67 v77.34,52.2 | v237.74,11.05 237.74,15.24 | v188.59,33.91 v188.59,10.67
YEND11  (via drill 0.35)
  Top 0.381: v93.34,43.43 92.96,43.81 78.87,43.81 73.15,49.53 2G.9 | 9H.9 222.88,13.72 221.74,12.57 187.07,12.57 184.4,9.91 164.21,9.91 v163.83,9.52 162.69,8.38 139.06,8.38 136.4,11.05 101.35,11.05 99.06,13.34 97.16,13.34 v95.25,15.24 | v228.22,31.62 235.46,31.62 10H.1
  Top 0.432: 1G.12 2G.9
  Bottom 0.381: v93.34,43.43 3H.1 93.34,31.62 95.25,29.72 v95.25,15.24 | v163.83,9.52 163.83,15.24 160.78,15.24 160.02,16 160.02,28.19 161.16,28.19 161.93,28.96 6H.15 | v228.22,31.62 225.93,29.34 225.93,14.86 225.17,14.1 222.88,14.1 9H.9
YOUT
  Top 0.381: VR2.3 315.47,64.77 313.18,64.77 VR2.2
  Bottom 0.381: IC15.1 313.18,57.15 313.18,64.39 VR2.2 313.18,64.77 313.18,73.53 314.33,74.68 C54.1 314.33,75.06 315.85,76.58 315.85,81.53 315.47,81.91 315.47,120.78 317.75,120.78 319.28,122.3 X1.4
YRATE  (via drill 0.35)
  Top 0.381: v168.4,240.03 180.21,240.03 180.21,238.12 182.12,236.22 7B.11 | v216.41,112.78 v169.55,112.78
  Bottom 0.381: 9H.14 220.98,28.58 220.98,44.96 224.79,48.77 224.79,60.2 222.88,62.1 | 220.22,96.77 222.12,96.77 222.88,97.54 9F.14 | 220.22,96.77 220.22,64.77 222.88,62.1 | 222.88,62.1 9G.14 | v168.4,240.03 168.4,131.83 169.55,130.68 v169.55,112.78 | v216.41,112.78 216.79,112.4 216.79,104.01 220.22,100.58 220.22,96.77
ZLD  (via drill 0.35)
  Top 0.381: 1H.11 58.29,10.67 v30.1,10.67 | v83.06,250.32 v30.1,250.32 | 3A.3 v83.06,274.32
  Bottom 0.381: v30.1,250.32 v30.1,10.67 | v83.06,274.32 v83.06,250.32
ZOUT
  Bottom 0.381: R24.2 T2.3 318.13,20.57 322.71,25.15 322.71,111.63 319.66,114.68 X1.2

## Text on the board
tPlace: Power Supply | -15V | -8V | +8V | +15V | +5V / LOGIC | 5V / DAC | Note: The analog circuits on this board / were NOT designed by Kincaid Arcade; / they were copied from the Atari Asteroids / Deluxe Manual. This project is intended / ONLY as a hobbyist's attempt to make a / vector arcade game, and neither Alexander / Haley nor Kincaid Arcade claim copyright or / ownership on any of the analog circuits. | A | Kincaid Arcade / Vector Graphics Card / REV - B | 8 | 1 | 2 | 3 | 4 | 5 | 6 | 7 | 8 | 9 | (c) Kincaid Arcade / 6/10/2020 / KincaidArcade.com | Power Input | Digital Circuits / Designed By: | B | 1 | Alexander K. Haley / (A 17 year old!) | 10 | C | X Analog Circuitry | D | X Gain | Sample & Hold | 6 | E | To Monitor | 1 | F | Y Analog Circuitry | Y Gain | G | All of the digital circuits in this design are licensed / under the Creative Commons License / CC BY-SA 4.0 | https://creativecommons.org/licenses/by-sa/4.0/ | H | Z-Amp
